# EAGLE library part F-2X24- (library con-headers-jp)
FEMALE HEADER
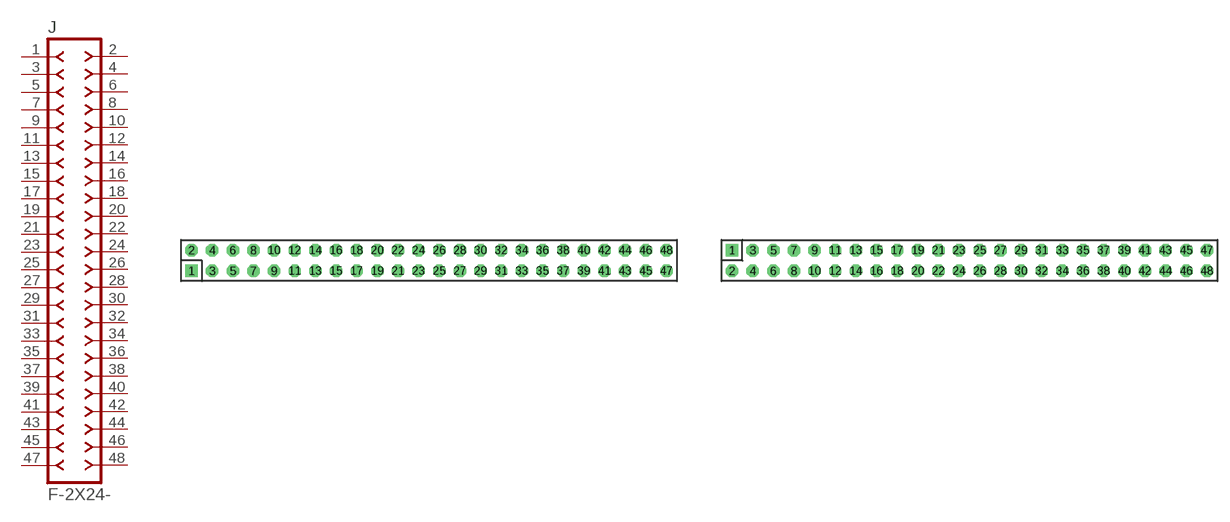
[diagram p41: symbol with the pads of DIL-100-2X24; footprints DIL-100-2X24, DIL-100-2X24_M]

Designator prefix J

## F-2X24-DIL-100  [DIL-100-2X24]
1  1  pas
2  2  pas
3  3  pas
4  4  pas
5  5  pas
6  6  pas
7  7  pas
8  8  pas
9  9  pas
10  10  pas
11  11  pas
12  12  pas
13  13  pas
14  14  pas
15  15  pas
16  16  pas
17  17  pas
18  18  pas
19  19  pas
20  20  pas
21  21  pas
22  22  pas
23  23  pas
24  24  pas
25  25  pas
26  26  pas
27  27  pas
28  28  pas
29  29  pas
30  30  pas
31  31  pas
32  32  pas
33  33  pas
34  34  pas
35  35  pas
36  36  pas
37  37  pas
38  38  pas
39  39  pas
40  40  pas
41  41  pas
42  42  pas
43  43  pas
44  44  pas
45  45  pas
46  46  pas
47  47  pas
48  48  pas

## F-2X24-DIL-100_M  [DIL-100-2X24_M]
Pads as for DIL-100-2X24

## F-2X24-DIL-2MM  [DIL-2MM-2X24]
Pads as for DIL-100-2X24

## F-2X24-DIL-2MM_M  [DIL-2MM-2X24_M]
Pads as for DIL-100-2X24

## Footprint DIL-100-2X24 (pad centres in mm)
PIN HEADER - 0.1"
drill 1.016 square: 1 -29.21,-1.27
drill 1.016 octagon: 2 -29.21,1.27; 3 -26.67,-1.27; 4 -26.67,1.27; 5 -24.13,-1.27; 6 -24.13,1.27; 7 -21.59,-1.27; 8 -21.59,1.27; 9 -19.05,-1.27; 10 -19.05,1.27; 11 -16.51,-1.27; 12 -16.51,1.27; 13 -13.97,-1.27; 14 -13.97,1.27; 15 -11.43,-1.27; 16 -11.43,1.27; 17 -8.89,-1.27; 18 -8.89,1.27; 19 -6.35,-1.27; 20 -6.35,1.27; 21 -3.81,-1.27; 22 -3.81,1.27; 23 -1.27,-1.27; 24 -1.27,1.27; 25 1.27,-1.27; 26 1.27,1.27; 27 3.81,-1.27; 28 3.81,1.27; 29 6.35,-1.27; 30 6.35,1.27; 31 8.89,-1.27; 32 8.89,1.27; 33 11.43,-1.27; 34 11.43,1.27; 35 13.97,-1.27; 36 13.97,1.27; 37 16.51,-1.27; 38 16.51,1.27; 39 19.05,-1.27; 40 19.05,1.27; 41 21.59,-1.27; 42 21.59,1.27; 43 24.13,-1.27; 44 24.13,1.27; 45 26.67,-1.27; 46 26.67,1.27; 47 29.21,-1.27; 48 29.21,1.27

## Footprint DIL-100-2X24_M (pad centres in mm)
PIN HEADER - MIRRORED 0.1"
drill 1.016 square: 1 -29.21,1.27
drill 1.016 octagon: 2 -29.21,-1.27; 3 -26.67,1.27; 4 -26.67,-1.27; 5 -24.13,1.27; 6 -24.13,-1.27; 7 -21.59,1.27; 8 -21.59,-1.27; 9 -19.05,1.27; 10 -19.05,-1.27; 11 -16.51,1.27; 12 -16.51,-1.27; 13 -13.97,1.27; 14 -13.97,-1.27; 15 -11.43,1.27; 16 -11.43,-1.27; 17 -8.89,1.27; 18 -8.89,-1.27; 19 -6.35,1.27; 20 -6.35,-1.27; 21 -3.81,1.27; 22 -3.81,-1.27; 23 -1.27,1.27; 24 -1.27,-1.27; 25 1.27,1.27; 26 1.27,-1.27; 27 3.81,1.27; 28 3.81,-1.27; 29 6.35,1.27; 30 6.35,-1.27; 31 8.89,1.27; 32 8.89,-1.27; 33 11.43,1.27; 34 11.43,-1.27; 35 13.97,1.27; 36 13.97,-1.27; 37 16.51,1.27; 38 16.51,-1.27; 39 19.05,1.27; 40 19.05,-1.27; 41 21.59,1.27; 42 21.59,-1.27; 43 24.13,1.27; 44 24.13,-1.27; 45 26.67,1.27; 46 26.67,-1.27; 47 29.21,1.27; 48 29.21,-1.27

## Footprint DIL-2MM-2X24 (pad centres in mm)
PIN HEADER - 2MM
drill 0.711 square: 1 -23,-1
drill 0.711: 2 -23,1; 3 -21,-1; 4 -21,1; 5 -19,-1; 6 -19,1; 7 -17,-1; 8 -17,1; 9 -15,-1; 10 -15,1; 11 -13,-1; 12 -13,1; 13 -11,-1; 14 -11,1; 15 -9,-1; 16 -9,1; 17 -7,-1; 18 -7,1; 19 -5,-1; 20 -5,1; 21 -3,-1; 22 -3,1; 23 -1,-1; 24 -1,1; 25 1,-1; 26 1,1; 27 3,-1; 28 3,1; 29 5,-1; 30 5,1; 31 7,-1; 32 7,1; 33 9,1; 34 9,-1; 35 11,1; 36 11,-1; 37 13,1; 38 13,-1; 39 15,1; 40 15,-1; 41 17,-1; 42 17,1; 43 19,-1; 44 19,1; 45 21,1; 46 21,-1; 47 23,1; 48 23,-1

## Footprint DIL-2MM-2X24_M (pad centres in mm)
PIN HEADER - MIRRORED 2MM
drill 0.711 square: 1 -23,1
drill 0.711: 2 -23,-1; 3 -21,1; 4 -21,-1; 5 -19,1; 6 -19,-1; 7 -17,1; 8 -17,-1; 9 -15,1; 10 -15,-1; 11 -13,1; 12 -13,-1; 13 -11,1; 14 -11,-1; 15 -9,1; 16 -9,-1; 17 -7,1; 18 -7,-1; 19 -5,1; 20 -5,-1; 21 -3,1; 22 -3,-1; 23 -1,1; 24 -1,-1; 25 1,1; 26 1,-1; 27 3,1; 28 3,-1; 29 5,1; 30 5,-1; 31 7,1; 32 7,-1; 33 9,-1; 34 9,1; 35 11,-1; 36 11,1; 37 13,-1; 38 13,1; 39 15,-1; 40 15,1; 41 17,1; 42 17,-1; 43 19,1; 44 19,-1; 45 21,-1; 46 21,1; 47 23,-1; 48 23,1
